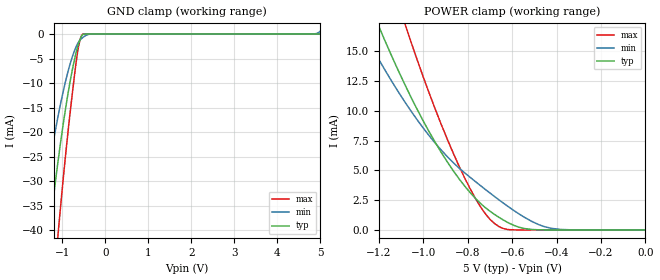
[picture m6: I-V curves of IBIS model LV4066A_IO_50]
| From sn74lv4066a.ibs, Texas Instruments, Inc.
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[Model]   LV4066A_IO_50
Model_type  Terminator
| variable   typ   min   max
C_comp   6.60pF   6.04pF   7.03pF
| C_tri-state   6.60pF   6.04pF   7.03pF
[Temperature Range]   40   100   -40
| Ambient temperature   25   85   -40
[Voltage range]   5   4.5   5.5
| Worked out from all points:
|   GND clamp passes 1 mA (typ) near -0.59 V on its own axis
|   POWER clamp passes 1 mA (typ) near -0.65 V on its own axis
[GND Clamp]
| LV4066A_IO_50
|   Voltage   I(typ)   I(min)   I(max)
-5V       -448.6mA   -321.8mA   -636mA
-1.55V    -60.17mA   -40.6mA    -90.41mA
-1.295V   -39.65mA   -26.21mA   -60.89mA
-1.11V    -26.47mA   -17.15mA   -41.62mA
-1.065V   -23.52mA   -15.15mA   -37.25mA
-880mV    -12.66mA   -7.986mA   -20.77mA
-685mV    -3.914mA   -2.681mA   -6.021mA
-600mV    -1.323mA   -1.343mA   -1.534mA
-525mV    -116.7uA   -717.4uA   -33.11uA
-310mV    -62.35nA   -7.607uA   -2.827nA
4.8V      106pA      3.758uA    73.35pA
5V        121.7pA    612.2uA    88.56pA
[POWER Clamp]
| LV4066A_IO_50
|   Voltage   I(typ)   I(min)   I(max)
-5V       323.9mA    250.8mA    425.6mA
-1.27V    20.3mA     16.69mA    28.82mA
-1.205V   17.32mA    14.49mA    24.64mA
-1.175V   16.01mA    13.52mA    22.78mA
-1.085V   12.3mA     10.81mA    17.46mA
-1.055V   11.15mA    9.985mA    15.79mA
-840mV    4.326mA    5.221mA    5.412mA
-740mV    2.191mA    3.69mA     1.878mA
-680mV    1.318mA    2.821mA    552.6uA
-570mV    236.4uA    1.36mA     3.237uA
-425mV    1.845uA    141.8uA    9.816nA
-84.45fV  121.7pA    639.6pA    126.6pA
